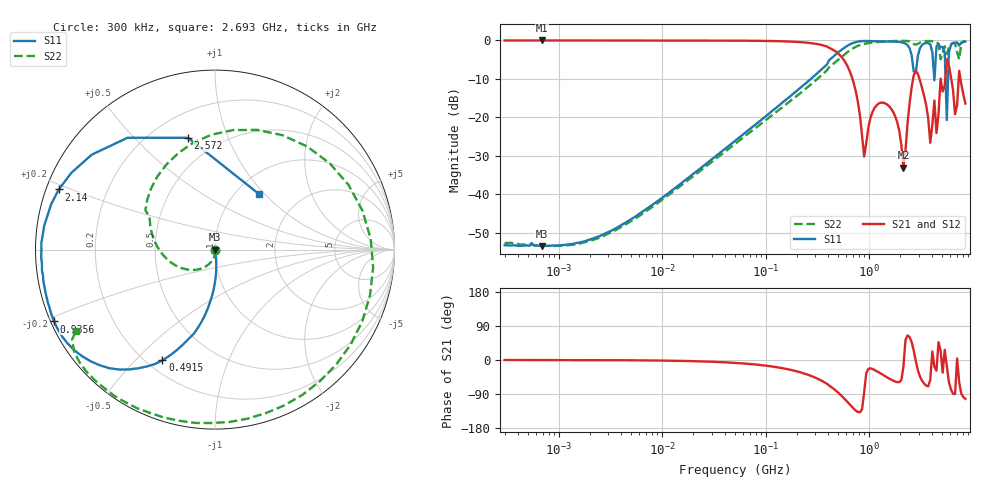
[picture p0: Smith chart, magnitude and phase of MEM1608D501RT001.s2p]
! S-Parameter Data Generated by TDK Corporation
! Copyright(C) 2025 TDK Corporation.
! All Rights Reserved.
! TDK P/N: MEM1608D501RT001 (3-terminal Filter)
! Property: Fc=500MHz
! Size(LxWxT): 1.6x0.8x0.6mm
! Model Type: s2p (Touchstone File Format Version 1.0)
! Frequency: DC=Yes Start=0.3MHz Stop=8500MHz 225points Log-sweep
! Model Generated on Feb. 6, 2025
! Terms and conditions regarding TDK Simulation Models:
! 1)This simulation model is being provided solely for informational
!  purposes. Please refer to the specifications of the products in
!  terms of detailed characteristics of such products.
! 2)In no event shall TDK Corporation of any of its subsidiaries be
!  liable for any loss or damage arising, directly or indirectly,
!  from any information contained in this simulation model, including,
!  but not limited to loss or damages arising from any inaccuracies,
!  omissions or errors in connection with such information.
! 3)Any and all copyrights on this simulation model are owned by
!  TDK Corporation.  Duplication or redistribution of this simulation
!  model without prior written permission from TDK Corporation
!  is prohibited.
! 4)This simulation model is subject to any modification or change
!  without any prior notice.
! 5)Neither TDK Corporation nor any of its subsidiaries shall make any
!  warranty, express or implied, including but not limited to the
!  correctness, implied warranties of merchantability and fitness for
!  a particular purpose with respect to this simulation models.
! 6)The use of this simulation model shall be deemed to have consented
!  to the terms and conditions hereof.
! Port Assignments:
!  1 ---@@@--- 2
! Applicable Conditions:
!  Temperature = 25 degC
!  DC Bias Current = 0 A
!  DC Bias Voltage = 0 V
!  Small Signal Operation
# Hz S MA R 50
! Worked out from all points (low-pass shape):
!   224 points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, 300 kHz to 8.5 GHz, reference 50 ohm
!   highest |S21| = -0.02 dB at 686.3 kHz (marker M1); lowest = -33.1 dB at 2.14 GHz (marker M2)
!   |S21| within 3 dB of the highest: start of sweep to 481 MHz
!   lowest |S11| = -53.6 dB at 686.3 kHz (marker M3), VSWR 1.00, Z = 50.2 - j0.0701 ohm
!   |S11| at or under -10 dB: start of sweep to 273.7 MHz; 4.254475 GHz to 4.274477 GHz (20 MHz wide, 0.469 % of centre); 5.465 GHz to 5.781 GHz (316.4 MHz wide, 5.63 % of centre)
!   |S22| runs from -53.5 to -0.1 dB; largest |S21 - S12| = 0.0037
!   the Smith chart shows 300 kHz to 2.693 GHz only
!   S11 on the Smith chart (normalised r, x): 300 kHz: 1.00, -0.00; 491.5 MHz: 0.26, -0.60; 935.6 MHz: 0.01, -0.21; 2.14 GHz: 0.04, +0.19; 2.572 GHz: 0.35, +0.73; 2.693 GHz: 1.26, +0.93
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300000  0.002165 -3.5  0.9976 -0.0  0.9978 0.2  0.002278 -10.1
686277.2  0.002101 -19.4  0.9982 -0.1  0.9973 0.1  0.002122 -20.4
1721110  0.002411 -38.6  0.9978 -0.3  0.9978 -0.1  0.002341 -37.5
9430415  0.008468 -73.2  0.9975 -1.4  0.9974 -1.3  0.007956 -76.5
5.167171e7  0.05048 -83.1  0.9925 -7.7  0.9925 -7.6  0.04626 -98.5
2.831228e8  0.3294 -96.9  0.916 -43.5  0.9162 -43.4  0.278 -170.3
4.915417e8  0.6831 -115.4  0.6911 -83.9  0.6911 -83.8  0.5458 119.7
9.355712e8  0.9823 -155.9  0.04548 -35.3  0.04562 -35.1  0.9126 -25.9
1.551304e9  0.9693 -177.4  0.1396 -48.7  0.1399 -48.5  0.9741 -101.8
2.140204e9  0.9325 158.9  0.0221 -18.2  0.02213 -18.5  0.9887 -132.7
2.572272e9  0.6402 103.5  0.2462 47.0  0.2464 47.2  0.9418 -147.8
2.693286e9  0.3948 51.9  0.3525 24.9  0.3527 25.0  0.8984 -149.7
2.952659e9  0.6306 -106.4  0.3665 -26.9  0.3665 -26.9  0.9032 -148.5
3.890506e9  0.8905 165.7  0.04658 -52.0  0.04654 -52.0  0.9816 -166.1
4.265177e9  0.3017 -136.6  0.1654 -18.2  0.1655 -18.3  0.9479 -173.6
4.465833e9  0.8323 -165.4  0.06232 -28.3  0.0624 -28.2  0.9521 -179.5
5.367404e9  0.6894 128.4  0.2582 26.7  0.2582 26.8  0.8398 -176.1
5.619915e9  0.09187 -58.2  0.5692 -15.1  0.57 -15.1  0.6655 -177.7
5.884306e9  0.6948 -144.8  0.4757 -57.3  0.4758 -57.5  0.8051 -172.8
7.072242e9  0.9407 165.2  0.1451 4.1  0.1451 4.2  0.6979 124.2
7.404957e9  0.8578 167.5  0.4021 -58.9  0.4025 -58.9  0.5682 -141.3
8.5e9  0.9639 153.3  0.1506 -102.5  0.1509 -103.1  0.9846 173.7
